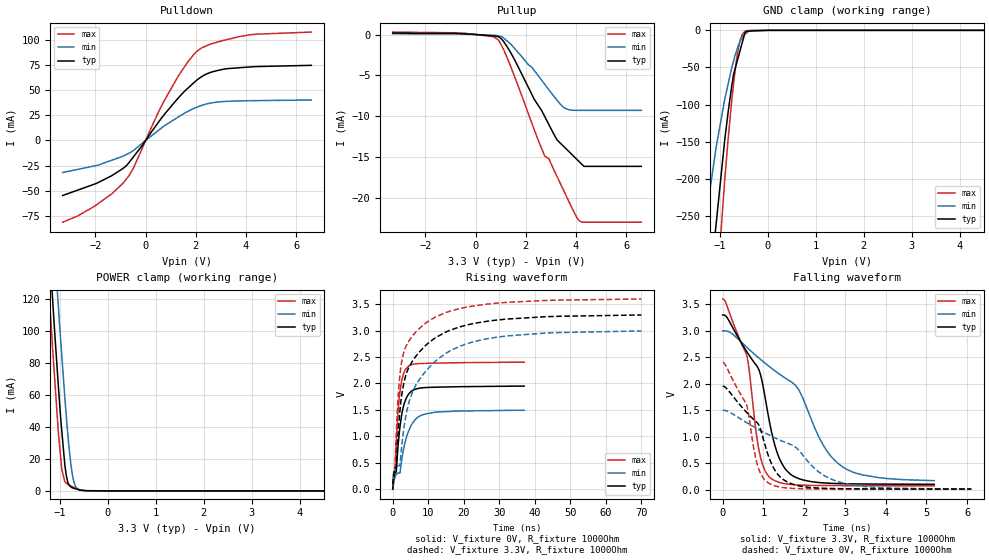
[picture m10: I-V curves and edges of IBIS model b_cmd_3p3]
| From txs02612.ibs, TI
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|   b_cmd_3p3 Model
[Model]   b_cmd_3p3
Model_type   I/O
Polarity   Non-Inverting
Enable   Active-High
Vinl = 0.15
Vinh = 3.1
Vmeas = 1.65
Vref = 1.65
Cref = 2pF
Rref = 1000
|   typ   min   max
|   (nom PVT)   (fast PVT)   (slow PVT)
|C_comp from frequency sweep method (F=30MHz)
C_comp   8.905e-12   8.807e-12   9.007e-12
|ON state : BUFFER OUTPUT TURNED HIGH
|C_comp   8.574e-12   8.419e-12   8.820e-12
|OFF state: BUFFER IN HIGH IMPEDANCE
|C_comp   8.905e-12   8.807e-12   9.007e-12
|C_comp from LC tank measurement(L=1nH)
|Average
|Resonant Frequency(Hz)   1.775e+09   1.785e+09   1.765e+09
|C_comp   8.048e-12   7.958e-12   8.139e-12
|ON state : BUFFER OUTPUT TURNED HIGH
|Resonant Frequency(Hz)   1.780e+09   1.790e+09   1.770e+09
|C_comp   8.003e-12   7.913e-12   8.093e-12
|OFF state: BUFFER IN HIGH IMPEDANCE
|Resonant Frequency(Hz)   1.770e+09   1.780e+09   1.760e+09
|C_comp   8.093e-12   8.003e-12   8.186e-12
[Model spec]
|subparameter
Vinl   0.15   0.15   0.15
Vinh   3.1   2.8   3.4
| Where nom  PVT is Nominal Process, 3.3V, 27C
|   Fast PVT is Strong Process,  3.6V, -40C
|   Slow PVT is Weak Process,   3V, 125C
[Voltage Range]   3.3   3   3.6
|Ambient Temperature   25   85   -40
|Junction Temperature
[Temperature Range]   27   125   -40
[Pullup Reference]   3.3   3   3.6
[Pulldown Reference]   0   0   0
[Power Clamp Reference]   3.3   3   3.6
[GND Clamp Reference]   0   0   0
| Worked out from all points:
|   slope of the pulldown table from 0 to 0.495 V, typ, clamps not added: 28.2 ohm
|   slope of the pullup table from 0 to 0.495 V, typ, clamps not added: 4.1 kohm
|   GND clamp passes 1 mA (typ) near -0.38 V on its own axis
|   POWER clamp passes 1 mA (typ) near -0.64 V on its own axis
|   falling waveform, V_fixture 3.3V, R_fixture 1000Ohm: 20-80 % time 772ps typ, 1.58ns min, 496ps max; typ from 3.3 V to 0.101 V
|   rising waveform, V_fixture 0V, R_fixture 1000Ohm: 20-80 % time 1.93ns typ, 3.73ns min, 1.45ns max; typ from 0.003 V to 1.95 V
|   rising waveform, V_fixture 3.3V, R_fixture 1000Ohm: 20-80 % time 7.06ns typ, 9.65ns min, 4.61ns max; typ from 0.09 V to 3.29 V
|   falling waveform, V_fixture 0V, R_fixture 1000Ohm: 20-80 % time 793ps typ, 1.68ns min, 498ps max; typ from 1.95 V to 0.01 V
[Pulldown]
|   Voltage   I(typ)   I(min)   I(max)
-3.3V     -54.75mA   -31.87mA   -81.33mA
-2.045V   -43.53mA   -25.39mA   -65.63mA
-1.346V   -35.04mA   -19.67mA   -53.15mA
-669.6mV  -22.25mA   -12.74mA   -35.38mA
-439.2mV  -14.85mA   -9.074mA   -24.99mA
723.6mV   25.17mA    14.07mA    38.7mA
1.246V    40.71mA    22.47mA    61.65mA
1.674V    51.79mA    28.84mA    77.9mA
2.167V    62.44mA    34.32mA    91.12mA
2.871V    69.7mA     38.26mA    98.03mA
4.162V    73.18mA    39.57mA    105.2mA
6.6V      74.78mA    40.27mA    107.9mA
[GND Clamp]
|   Voltage   I(typ)   I(min)   I(max)
-3.3V     -2.627A    -1.685A    -3.329A
-1.343V   -460.3mA   -275.9mA   -644.7mA
-1.285V   -415.7mA   -250mA     -579.4mA
-1.08V    -262.1mA   -158.2mA   -364.2mA
-897.6mV  -146.8mA   -92.53mA   -200.6mA
-745.8mV  -72.3mA    -48.84mA   -90.86mA
-662.4mV  -46.98mA   -29.86mA   -43.92mA
-615.6mV  -35.94mA   -20.72mA   -24.65mA
-532.8mV  -16.4mA    -9.37mA    -5.477mA
-475.2mV  -2.809mA   -5.07mA    -1.318mA
-285mV    -754uA     -123uA     -75.81uA
6.6V      0A         0A         0A
[Pullup]
|   Voltage   I(typ)   I(min)   I(max)
-3.3V     174.2uA    84.77uA    295.6uA
-439.2mV  75.72uA    53.37uA    157.4uA
910.8mV   -276.4uA   -150.6uA   -666.9uA
1.386V    -2.149mA   -1.119mA   -3.808mA
2.32V     -7.823mA   -4.322mA   -11.48mA
2.747V    -9.975mA   -6.053mA   -14.8mA
2.912V    -10.96mA   -6.726mA   -15.15mA
3.241V    -12.86mA   -8.003mA   -17.32mA
3.549V    -13.79mA   -8.986mA   -19.32mA
4.061V    -15.33mA   -9.26mA    -22.51mA
4.316V    -16.1mA    -9.26mA    -22.92mA
6.6V      -16.1mA    -9.26mA    -22.92mA
[POWER Clamp]
|   Voltage   I(typ)   I(min)   I(max)
-3.3V     1.217A     1.246A     1.197A
-1.287V   183.5mA    233.1mA    154.4mA
-1.161V   124.1mA    173.8mA    93.5mA
-1.152V   119.9mA    169.6mA    89.15mA
-1.033V   66.1mA     115.9mA    37.16mA
-961.2mV  37.89mA    85.1mA     13.73mA
-867.9mV  9.882mA    47.42mA    5.033mA
-810mV    3.871mA    27.49mA    3.682mA
-745.8mV  2.006mA    11.29mA    2.712mA
-645mV    1.081mA    1.672mA    1.329mA
-432mV    168.8uA    75.14uA    48.52uA
6.6V      0A         0A         0A
[Ramp]
R_load = 1000
|   typ   min   max
dV/dt_r   1.17037/1.93139e-09   0.897496/3.72343e-09   1.44105/1.45356e-09
dV/dt_f   1.9258/7.72709e-10   1.71429/1.59609e-09   2.12121/4.96621e-10
[Falling Waveform]
V_fixture = 3.3V
V_fixture_min = 3V
V_fixture_max = 3.6V
R_fixture = 1000Ohm
|   Time   V(typ)   V(min)   V(max)
0s        3.3V       3V         3.6V
600ps     2.596V     2.683V     2.501V
900ps     2.24V      2.478V     706.8mV
1.175ns   1.173V     2.306V     218.1mV
1.4ns     572.9mV    2.178V     133.7mV
1.675ns   284mV      2.039V     97.14mV
1.9ns     199mV      1.837V     85.69mV
2.475ns   126.7mV    829.7mV    76.82mV
2.975ns   111.1mV    413.6mV    74.71mV
5.19ns    101.1mV    170.4mV    72.02mV
[Rising Waveform]
V_fixture = 0V
V_fixture_min = 0V
V_fixture_max = 0V
R_fixture = 1000Ohm
|   Time   V(typ)   V(min)   V(max)
0s        3.365mV    3.408mV    3.41mV
675ps     310.6mV    238.4mV    334.3mV
1ns       330mV      280.7mV    863.8mV
1.25ns    583.2mV    296.3mV    1.185V
1.95ns    1.125V     304.5mV    1.792V
2.875ns   1.527V     696.9mV    2.144V
4.2ns     1.771V     1.052V     2.313V
6.225ns   1.888V     1.31V      2.37V
9.3ns     1.924V     1.425V     2.38V
37ns      1.95V      1.494V     2.402V
[Rising Waveform]
V_fixture = 3.3V
V_fixture_min = 3V
V_fixture_max = 3.6V
R_fixture = 1000Ohm
|   Time   V(typ)   V(min)   V(max)
0s        90.17mV    142.5mV    64.56mV
675ps     399.8mV    379.9mV    407.1mV
1.025ns   443.3mV    422.9mV    1.078V
1.65ns    1.178V     445.9mV    1.877V
2.05ns    1.499V     471.3mV    2.176V
2.675ns   1.84V      906.1mV    2.466V
4.7ns     2.325V     1.676V     2.817V
9.15ns    2.712V     2.221V     3.134V
26.48ns   3.174V     2.844V     3.498V
69.98ns   3.293V     2.991V     3.595V
[Falling Waveform]
V_fixture = 0V
V_fixture_min = 0V
V_fixture_max = 0V
R_fixture = 1000Ohm
|   Time   V(typ)   V(min)   V(max)
0s        1.954V     1.5V       2.405V
575ps     1.469V     1.271V     1.628V
850ps     1.261V     1.147V     471.8mV
975ps     1.019V     1.095V     241mV
1.175ns   529.2mV    1.017V     103.3mV
1.4ns     246.9mV    936.4mV    48.76mV
1.675ns   113.7mV    851.6mV    25.08mV
2.35ns    29.33mV    338.6mV    12.54mV
2.925ns   16.69mV    129.8mV    10.53mV
6.1ns     9.674mV    13.75mV    8.287mV
